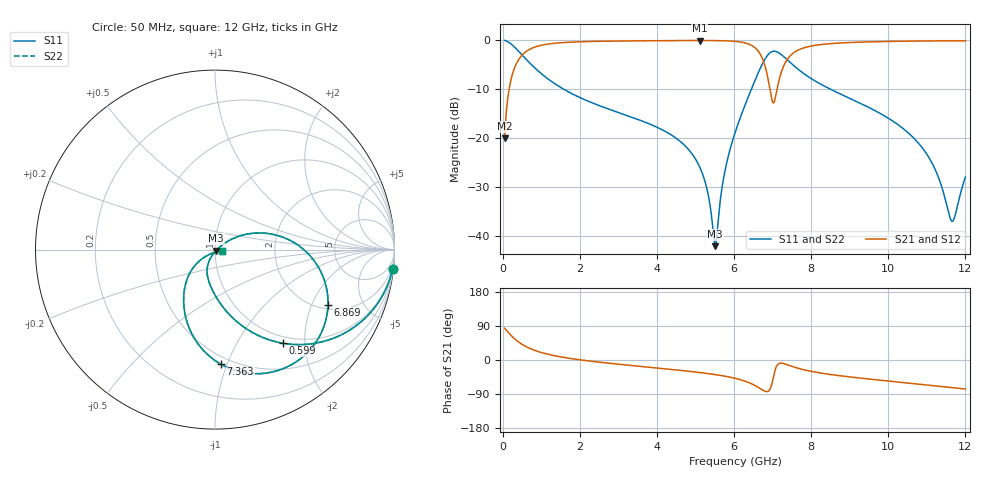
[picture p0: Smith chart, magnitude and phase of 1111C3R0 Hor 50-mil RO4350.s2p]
# GHz S MA R 50
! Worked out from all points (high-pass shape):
!   11951 points, 50 MHz to 12 GHz, reference 50 ohm
!   highest |S21| = -0.05 dB at 5.107 GHz (marker M1); lowest = -20.0 dB at 50 MHz (marker M2)
!   |S21| within 3 dB of the highest: 501.2 MHz to 6.695 GHz (6.194 GHz wide, 172 % of centre); 7.473 GHz to end of sweep
!   lowest |S11| = -42.1 dB at 5.512 GHz (marker M3), VSWR 1.02, Z = 50.6 - j0.536 ohm
!   |S11| at or under -10 dB: 1.579 GHz to 6.45 GHz (4.871 GHz wide, 121 % of centre); 8.495 GHz to end of sweep
!   |S22| runs from -42.1 to 0.0 dB; largest |S21 - S12| = 0
!   S11 on the Smith chart (normalised r, x): 50 MHz: 1, -19; 599 MHz: 0.89, -1.58; 6.869 GHz: 2.19, -2.65; 7.363 GHz: 0.44, -0.95; 12 GHz: 1.08, -0.01
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0.05  0.9949 -6.1  0.0995 83.9  0.0995 83.9  0.9949 -6.1
0.248  0.8953 -28.1  0.4427 61.7  0.4427 61.7  0.8953 -28.1
0.599  0.6443 -54.1  0.7627 35.7  0.7627 35.7  0.6443 -54.1
1.13  0.4147 -73.5  0.9085 16.3  0.9085 16.3  0.4147 -73.5
2.042  0.2552 -89.7  0.9656 -0.0  0.9656 -0.0  0.2552 -89.7
4.034  0.1271 -110.5  0.9895 -21.4  0.9895 -21.4  0.1271 -110.5
4.696  0.08579 -116.1  0.9928 -28.3  0.9928 -28.3  0.08579 -116.1
5.107  0.0507 -117.7  0.9937 -33.0  0.9937 -33.0  0.0507 -117.7
5.309  0.02876 -113.7  0.9934 -35.6  0.9934 -35.6  0.02876 -113.7
5.512  0.007825 -42.6  0.9919 -38.5  0.9919 -38.5  0.007825 -42.6
5.745  0.04197 32.0  0.9876 -42.4  0.9876 -42.4  0.04197 32.0
6.025  0.1128 31.8  0.974 -48.2  0.974 -48.2  0.1128 31.8
6.564  0.406 8.4  0.826 -68.5  0.826 -68.5  0.406 8.4
6.869  0.7011 -26.1  0.4262 -83.1  0.4262 -83.1  0.7011 -26.1
7.031  0.7722 -50.4  0.2302 -40.2  0.2302 -40.2  0.7722 -50.4
7.173  0.7389 -69.1  0.3984 -9.1  0.3984 -9.1  0.7389 -69.1
7.363  0.64 -87.0  0.6218 -11.8  0.6218 -11.8  0.64 -87.0
8.017  0.4016 -114.4  0.8751 -30.3  0.8751 -30.3  0.4016 -114.4
10.009  0.1587 -140.2  0.9721 -55.6  0.9721 -55.6  0.1587 -140.2
11.034  0.06497 -143.9  0.9836 -66.2  0.9836 -66.2  0.06497 -143.9
11.643  0.01412 -79.8  0.9855 -72.7  0.9855 -72.7  0.01412 -79.8
12  0.03986 -7.5  0.9846 -76.6  0.9846 -76.6  0.03986 -7.5
